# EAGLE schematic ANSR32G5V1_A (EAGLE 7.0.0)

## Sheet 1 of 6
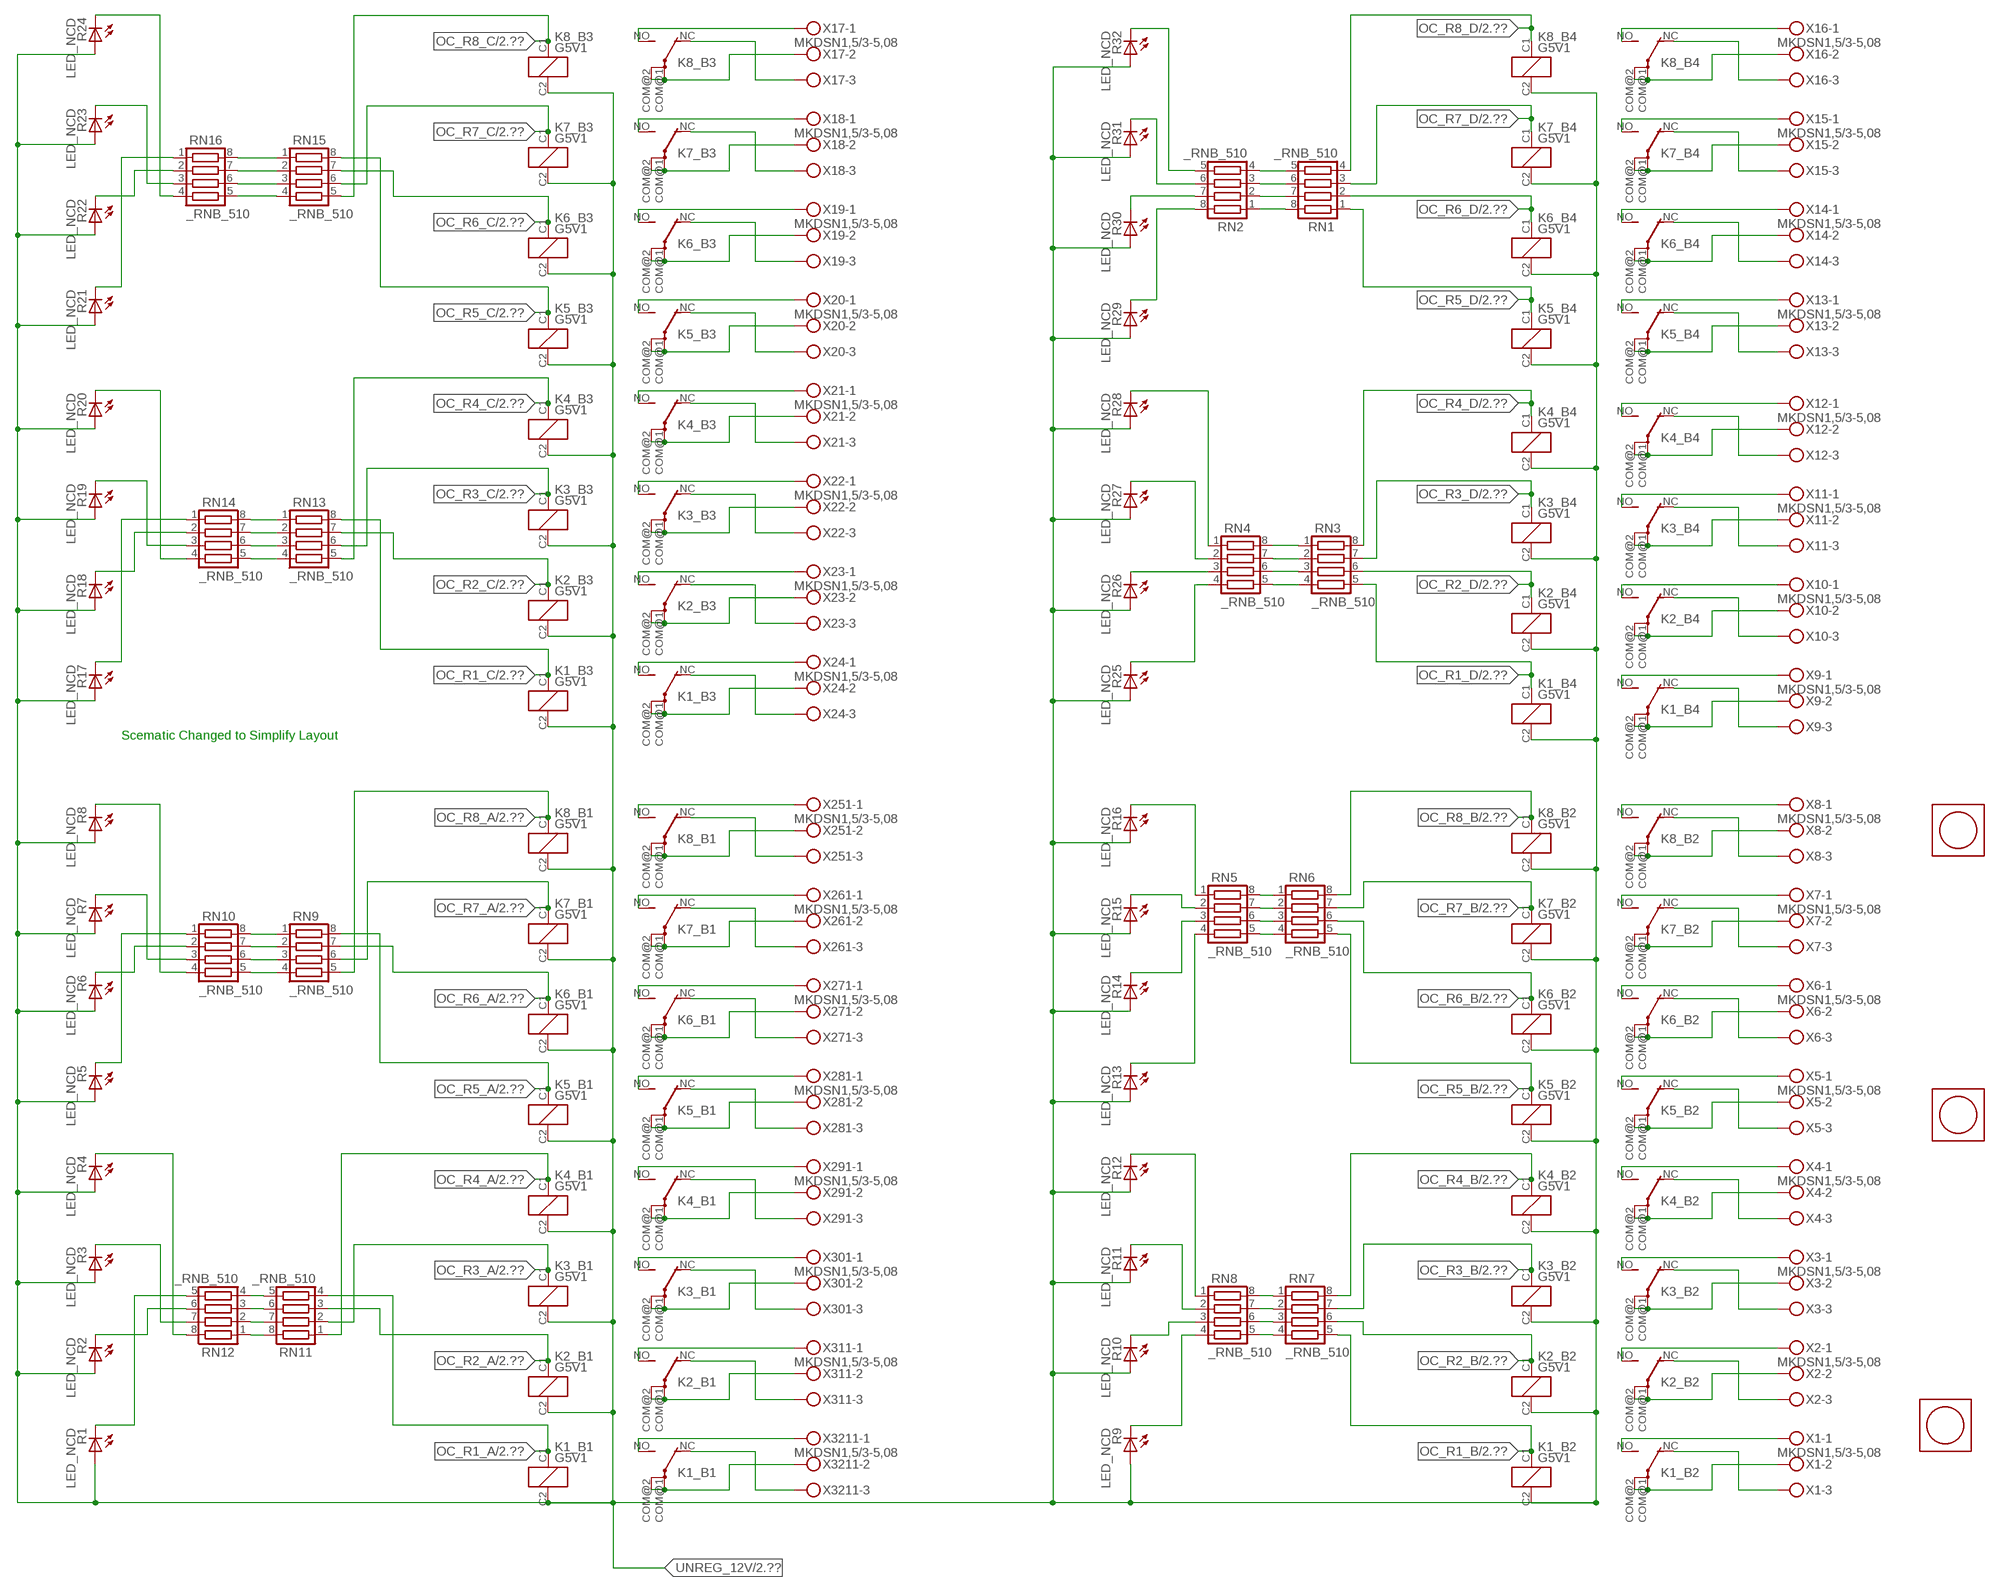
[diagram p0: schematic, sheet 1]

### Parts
K1_B1  G5V1  [G5V1]
K1_B2  G5V1  [G5V1]
K1_B3  G5V1  [G5V1]
K1_B4  G5V1  [G5V1]
K2_B1  G5V1  [G5V1]
K2_B2  G5V1  [G5V1]
K2_B3  G5V1  [G5V1]
K2_B4  G5V1  [G5V1]
K3_B1  G5V1  [G5V1]
K3_B2  G5V1  [G5V1]
K3_B3  G5V1  [G5V1]
K3_B4  G5V1  [G5V1]
K4_B1  G5V1  [G5V1]
K4_B2  G5V1  [G5V1]
K4_B3  G5V1  [G5V1]
K4_B4  G5V1  [G5V1]
K5_B1  G5V1  [G5V1]
K5_B2  G5V1  [G5V1]
K5_B3  G5V1  [G5V1]
K5_B4  G5V1  [G5V1]
K6_B1  G5V1  [G5V1]
K6_B2  G5V1  [G5V1]
K6_B3  G5V1  [G5V1]
K6_B4  G5V1  [G5V1]
K7_B1  G5V1  [G5V1]
K7_B2  G5V1  [G5V1]
K7_B3  G5V1  [G5V1]
K7_B4  G5V1  [G5V1]
K8_B1  G5V1  [G5V1]
K8_B2  G5V1  [G5V1]
K8_B3  G5V1  [G5V1]
K8_B4  G5V1  [G5V1]
R1  LED_NCD  [CHIPLED_0603]
R2  LED_NCD  [CHIPLED_0603]
R3  LED_NCD  [CHIPLED_0603]
R4  LED_NCD  [CHIPLED_0603]
R5  LED_NCD  [CHIPLED_0603]
R6  LED_NCD  [CHIPLED_0603]
R7  LED_NCD  [CHIPLED_0603]
R8  LED_NCD  [CHIPLED_0603]
R9  LED_NCD  [CHIPLED_0603]
R10  LED_NCD  [CHIPLED_0603]
R11  LED_NCD  [CHIPLED_0603]
R12  LED_NCD  [CHIPLED_0603]
R13  LED_NCD  [CHIPLED_0603]
R14  LED_NCD  [CHIPLED_0603]
R15  LED_NCD  [CHIPLED_0603]
R16  LED_NCD  [CHIPLED_0603]
R17  LED_NCD  [CHIPLED_0603]
R18  LED_NCD  [CHIPLED_0603]
R19  LED_NCD  [CHIPLED_0603]
R20  LED_NCD  [CHIPLED_0603]
R21  LED_NCD  [CHIPLED_0603]
R22  LED_NCD  [CHIPLED_0603]
R23  LED_NCD  [CHIPLED_0603]
R24  LED_NCD  [CHIPLED_0603]
R25  LED_NCD  [CHIPLED_0603]
R26  LED_NCD  [CHIPLED_0603]
R27  LED_NCD  [CHIPLED_0603]
R28  LED_NCD  [CHIPLED_0603]
R29  LED_NCD  [CHIPLED_0603]
R30  LED_NCD  [CHIPLED_0603]
R31  LED_NCD  [CHIPLED_0603]
R32  LED_NCD  [CHIPLED_0603]
RN1  _RNB_510  [RNB]
RN2  _RNB_510  [RNB]
RN3  _RNB_510  [RNB]
RN4  _RNB_510  [RNB]
RN5  _RNB_510  [RNB]
RN6  _RNB_510  [RNB]
RN7  _RNB_510  [RNB]
RN8  _RNB_510  [RNB]
RN9  _RNB_510  [RNB]
RN10  _RNB_510  [RNB]
RN11  _RNB_510  [RNB]
RN12  _RNB_510  [RNB]
RN13  _RNB_510  [RNB]
RN14  _RNB_510  [RNB]
RN15  _RNB_510  [RNB]
RN16  _RNB_510  [RNB]
U$1  PCB_MOUNTING_HOLE  [PCB_MOUNTING_HOLE]
U$2  PCB_MOUNTING_HOLE  [PCB_MOUNTING_HOLE]
U$3  PCB_MOUNTING_HOLE  [PCB_MOUNTING_HOLE]
X1  MKDSN1,5/3-5,08  [MKDSN1,5/3-5,08]
X2  MKDSN1,5/3-5,08  [MKDSN1,5/3-5,08]
X3  MKDSN1,5/3-5,08  [MKDSN1,5/3-5,08]
X4  MKDSN1,5/3-5,08  [MKDSN1,5/3-5,08]
X5  MKDSN1,5/3-5,08  [MKDSN1,5/3-5,08]
X6  MKDSN1,5/3-5,08  [MKDSN1,5/3-5,08]
X7  MKDSN1,5/3-5,08  [MKDSN1,5/3-5,08]
X8  MKDSN1,5/3-5,08  [MKDSN1,5/3-5,08]
X9  MKDSN1,5/3-5,08  [MKDSN1,5/3-5,08]
X10  MKDSN1,5/3-5,08  [MKDSN1,5/3-5,08]
X11  MKDSN1,5/3-5,08  [MKDSN1,5/3-5,08]
X12  MKDSN1,5/3-5,08  [MKDSN1,5/3-5,08]
X13  MKDSN1,5/3-5,08  [MKDSN1,5/3-5,08]
X14  MKDSN1,5/3-5,08  [MKDSN1,5/3-5,08]
X15  MKDSN1,5/3-5,08  [MKDSN1,5/3-5,08]
X16  MKDSN1,5/3-5,08  [MKDSN1,5/3-5,08]
X17  MKDSN1,5/3-5,08  [MKDSN1,5/3-5,08]
X18  MKDSN1,5/3-5,08  [MKDSN1,5/3-5,08]
X19  MKDSN1,5/3-5,08  [MKDSN1,5/3-5,08]
X20  MKDSN1,5/3-5,08  [MKDSN1,5/3-5,08]
X21  MKDSN1,5/3-5,08  [MKDSN1,5/3-5,08]
X22  MKDSN1,5/3-5,08  [MKDSN1,5/3-5,08]
X23  MKDSN1,5/3-5,08  [MKDSN1,5/3-5,08]
X24  MKDSN1,5/3-5,08  [MKDSN1,5/3-5,08]
X251  MKDSN1,5/3-5,08  [MKDSN1,5/3-5,08]
X261  MKDSN1,5/3-5,08  [MKDSN1,5/3-5,08]
X271  MKDSN1,5/3-5,08  [MKDSN1,5/3-5,08]
X281  MKDSN1,5/3-5,08  [MKDSN1,5/3-5,08]
X291  MKDSN1,5/3-5,08  [MKDSN1,5/3-5,08]
X301  MKDSN1,5/3-5,08  [MKDSN1,5/3-5,08]
X311  MKDSN1,5/3-5,08  [MKDSN1,5/3-5,08]
X3211  MKDSN1,5/3-5,08  [MKDSN1,5/3-5,08]

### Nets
N$1: K8_B2.COM@1(2:P) K8_B2.COM@2(2:P) X8.2
N$2: K8_B2.NC(2:O) X8.3
N$3: K8_B2.NO(2:S) X8.1
N$4: K7_B2.NO(2:S) X7.1
N$5: K6_B2.NO(2:S) X6.1
N$6: K7_B2.NC(2:O) X7.3
N$7: K7_B2.COM@1(2:P) K7_B2.COM@2(2:P) X7.2
N$8: K6_B2.NC(2:O) X6.3
N$10: K4_B2.NO(2:S) X4.1
N$11: K4_B2.NC(2:O) X4.3
N$12: K4_B2.COM@1(2:P) K4_B2.COM@2(2:P) X4.2
N$14: K6_B2.COM@1(2:P) K6_B2.COM@2(2:P) X6.2
N$33: K5_B2.NC(2:O) X5.3
N$34: K5_B2.COM@1(2:P) K5_B2.COM@2(2:P) X5.2
N$35: K5_B2.NO(2:S) X5.1
N$36: K3_B2.NO(2:S) X3.1
N$37: K3_B2.NC(2:O) X3.3
N$38: K3_B2.COM@1(2:P) K3_B2.COM@2(2:P) X3.2
N$39: K2_B2.NO(2:S) X2.1
N$40: K2_B2.NC(2:O) X2.3
N$41: K2_B2.COM@1(2:P) K2_B2.COM@2(2:P) X2.2
N$42: K1_B2.NO(2:S) X1.1
N$43: K1_B2.NC(2:O) X1.3
N$44: K1_B2.COM@1(2:P) K1_B2.COM@2(2:P) X1.2
N$78: K1_B4.COM@1(2:P) K1_B4.COM@2(2:P) X9.2
N$79: K1_B4.NC(2:O) X9.3
N$80: K1_B4.NO(2:S) X9.1
N$81: K2_B4.NO(2:S) X10.1
N$82: K3_B4.NO(2:S) X11.1
N$83: K2_B4.NC(2:O) X10.3
N$84: K2_B4.COM@1(2:P) K2_B4.COM@2(2:P) X10.2
N$85: K3_B4.NC(2:O) X11.3
N$86: K3_B4.COM@1(2:P) K3_B4.COM@2(2:P) X11.2
N$87: K4_B4.NC(2:O) X12.3
N$88: K4_B4.COM@1(2:P) K4_B4.COM@2(2:P) X12.2
N$89: K4_B4.NO(2:S) X12.1
N$90: K5_B4.NO(2:S) X13.1
N$91: K5_B4.NC(2:O) X13.3
N$92: K5_B4.COM@1(2:P) K5_B4.COM@2(2:P) X13.2
N$93: K6_B4.NO(2:S) X14.1
N$94: K6_B4.NC(2:O) X14.3
N$95: K6_B4.COM@1(2:P) K6_B4.COM@2(2:P) X14.2
N$96: K7_B4.NO(2:S) X15.1
N$97: K7_B4.NC(2:O) X15.3
N$98: K7_B4.COM@1(2:P) K7_B4.COM@2(2:P) X15.2
N$99: K8_B4.NO(2:S) X16.1
N$100: K8_B4.NC(2:O) X16.3
N$101: K8_B4.COM@1(2:P) K8_B4.COM@2(2:P) X16.2
N$179: K8_B3.COM@1(2:P) K8_B3.COM@2(2:P) X17.2
N$180: K8_B3.NC(2:O) X17.3
N$181: K8_B3.NO(2:S) X17.1
N$182: K7_B3.NO(2:S) X18.1
N$183: K6_B3.NO(2:S) X19.1
N$184: K7_B3.NC(2:O) X18.3
N$185: K7_B3.COM@1(2:P) K7_B3.COM@2(2:P) X18.2
N$186: K6_B3.NC(2:O) X19.3
N$187: K6_B3.COM@1(2:P) K6_B3.COM@2(2:P) X19.2
N$188: K5_B3.NC(2:O) X20.3
N$189: K5_B3.COM@1(2:P) K5_B3.COM@2(2:P) X20.2
N$190: K5_B3.NO(2:S) X20.1
N$191: K4_B3.NO(2:S) X21.1
N$192: K4_B3.NC(2:O) X21.3
N$193: K4_B3.COM@1(2:P) K4_B3.COM@2(2:P) X21.2
N$194: K3_B3.NO(2:S) X22.1
N$195: K3_B3.NC(2:O) X22.3
N$196: K3_B3.COM@1(2:P) K3_B3.COM@2(2:P) X22.2
N$197: K2_B3.NO(2:S) X23.1
N$198: K2_B3.NC(2:O) X23.3
N$199: K2_B3.COM@1(2:P) K2_B3.COM@2(2:P) X23.2
N$200: K1_B3.NO(2:S) X24.1
N$201: K1_B3.NC(2:O) X24.3
N$202: K1_B3.COM@1(2:P) K1_B3.COM@2(2:P) X24.2
N$203: K8_B1.COM@1(2:P) K8_B1.COM@2(2:P) X251.2
N$204: K8_B1.NC(2:O) X251.3
N$205: K8_B1.NO(2:S) X251.1
N$206: K7_B1.NO(2:S) X261.1
N$207: K6_B1.NO(2:S) X271.1
N$208: K7_B1.NC(2:O) X261.3
N$209: K7_B1.COM@1(2:P) K7_B1.COM@2(2:P) X261.2
N$210: K6_B1.NC(2:O) X271.3
N$211: K6_B1.COM@1(2:P) K6_B1.COM@2(2:P) X271.2
N$212: K5_B1.NC(2:O) X281.3
N$213: K5_B1.COM@1(2:P) K5_B1.COM@2(2:P) X281.2
N$214: K5_B1.NO(2:S) X281.1
N$215: K4_B1.NO(2:S) X291.1
N$216: K4_B1.NC(2:O) X291.3
N$217: K4_B1.COM@1(2:P) K4_B1.COM@2(2:P) X291.2
N$218: K3_B1.NO(2:S) X301.1
N$219: K3_B1.NC(2:O) X301.3
N$220: K3_B1.COM@1(2:P) K3_B1.COM@2(2:P) X301.2
N$221: K2_B1.NO(2:S) X311.1
N$222: K2_B1.NC(2:O) X311.3
N$223: K2_B1.COM@1(2:P) K2_B1.COM@2(2:P) X311.2
N$224: K1_B1.NO(2:S) X3211.1
N$225: K1_B1.NC(2:O) X3211.3
N$226: K1_B1.COM@1(2:P) K1_B1.COM@2(2:P) X3211.2
N$440: R30.C RN2.7
N$441: R16.C RN5.1
N$442: RN7.2 RN8.7
N$443: RN7.3 RN8.6
N$444: RN7.4 RN8.5
N$445: R15.C RN5.2
N$446: R26.C RN4.3
N$447: R13.C RN5.4
N$448: RN5.5 RN6.4
N$449: RN7.1 RN8.8
N$450: R12.C RN8.1
N$451: RN5.6 RN6.3
N$452: R11.C RN8.2
N$453: RN5.7 RN6.2
N$454: RN5.8 RN6.1
N$455: RN3.4 RN4.5
N$456: R32.C RN2.5
N$458: R14.C RN5.3
N$459: R10.C RN8.3
N$460: R29.C RN2.8
N$461: R28.C RN4.1
N$462: R27.C RN4.2
N$463: RN11.5 RN12.4
N$464: R25.C RN4.4
N$465: RN1.8 RN2.1
N$466: RN1.7 RN2.2
N$467: RN1.6 RN2.3
N$468: RN1.5 RN2.4
N$469: R31.C RN2.6
N$470: R9.C RN8.4
N$473: R1.C RN12.5
N$474: RN11.6 RN12.3
N$475: R2.C RN12.6
N$476: R3.C RN12.7
N$477: RN9.4 RN10.5
N$478: RN9.3 RN10.6
N$479: RN9.2 RN10.7
N$480: RN9.1 RN10.8
N$481: RN11.7 RN12.2
N$482: R5.C RN10.1
N$483: R4.C RN12.8
N$484: R7.C RN10.3
N$485: R8.C RN10.4
N$486: R6.C RN10.2
N$487: R19.C RN14.3
N$488: R18.C RN14.2
N$489: R17.C RN14.1
N$490: R24.C RN16.4
N$491: RN15.3 RN16.6
N$492: RN15.2 RN16.7
N$493: RN15.1 RN16.8
N$494: R20.C RN14.4
N$495: R23.C RN16.3
N$496: R22.C RN16.2
N$497: R21.C RN16.1
N$500: RN11.8 RN12.1
N$501: RN13.4 RN14.5
N$502: RN13.3 RN14.6
N$503: RN13.2 RN14.7
N$504: RN13.1 RN14.8
N$505: RN3.3 RN4.6
N$506: RN3.2 RN4.7
N$507: RN3.1 RN4.8
N$514: RN15.4 RN16.5
OC_R1_A: K1_B1.C1(1:C1) RN11.4 ; also sheet 2
OC_R1_B: K1_B2.C1(1:C1) RN7.5 ; also sheet 2
OC_R1_C: K1_B3.C1(1:C1) RN13.8 ; also sheet 2
OC_R1_D: K1_B4.C1(1:C1) RN3.5 ; also sheet 2
OC_R2_A: K2_B1.C1(1:C1) RN11.3 ; also sheet 2
OC_R2_B: K2_B2.C1(1:C1) RN7.6 ; also sheet 2
OC_R2_C: K2_B3.C1(1:C1) RN13.7 ; also sheet 2
OC_R2_D: K2_B4.C1(1:C1) RN3.6 ; also sheet 2
OC_R3_A: K3_B1.C1(1:C1) RN11.2 ; also sheet 2
OC_R3_B: K3_B2.C1(1:C1) RN7.7 ; also sheet 2
OC_R3_C: K3_B3.C1(1:C1) RN13.6 ; also sheet 2
OC_R3_D: K3_B4.C1(1:C1) RN3.7 ; also sheet 2
OC_R4_A: K4_B1.C1(1:C1) RN11.1 ; also sheet 2
OC_R4_B: K4_B2.C1(1:C1) RN7.8 ; also sheet 2
OC_R4_C: K4_B3.C1(1:C1) RN13.5 ; also sheet 2
OC_R4_D: K4_B4.C1(1:C1) RN3.8 ; also sheet 2
OC_R5_A: K5_B1.C1(1:C1) RN9.8 ; also sheet 2
OC_R5_B: K5_B2.C1(1:C1) RN6.5 ; also sheet 2
OC_R5_C: K5_B3.C1(1:C1) RN15.8 ; also sheet 2
OC_R5_D: K5_B4.C1(1:C1) RN1.1 ; also sheet 2
OC_R6_A: K6_B1.C1(1:C1) RN9.7 ; also sheet 2
OC_R6_B: K6_B2.C1(1:C1) RN6.6 ; also sheet 2
OC_R6_C: K6_B3.C1(1:C1) RN15.7 ; also sheet 2
OC_R6_D: K6_B4.C1(1:C1) RN1.2 ; also sheet 2
OC_R7_A: K7_B1.C1(1:C1) RN9.6 ; also sheet 2
OC_R7_B: K7_B2.C1(1:C1) RN6.7 ; also sheet 2
OC_R7_C: K7_B3.C1(1:C1) RN15.6 ; also sheet 2
OC_R7_D: K7_B4.C1(1:C1) RN1.3 ; also sheet 2
OC_R8_A: K8_B1.C1(1:C1) RN9.5 ; also sheet 2
OC_R8_B: K8_B2.C1(1:C1) RN6.8 ; also sheet 2
OC_R8_C: K8_B3.C1(1:C1) RN15.5 ; also sheet 2
OC_R8_D: K8_B4.C1(1:C1) RN1.4 ; also sheet 2
UNREG_12V: K1_B1.C2(1:C2) K1_B2.C2(1:C2) K1_B3.C2(1:C2) K1_B4.C2(1:C2) K2_B1.C2(1:C2) K2_B2.C2(1:C2) K2_B3.C2(1:C2) K2_B4.C2(1:C2) K3_B1.C2(1:C2) K3_B2.C2(1:C2) K3_B3.C2(1:C2) K3_B4.C2(1:C2) K4_B1.C2(1:C2) K4_B2.C2(1:C2) K4_B3.C2(1:C2) K4_B4.C2(1:C2) K5_B1.C2(1:C2) K5_B2.C2(1:C2) K5_B3.C2(1:C2) K5_B4.C2(1:C2) K6_B1.C2(1:C2) K6_B2.C2(1:C2) K6_B3.C2(1:C2) K6_B4.C2(1:C2) K7_B1.C2(1:C2) K7_B2.C2(1:C2) K7_B3.C2(1:C2) K7_B4.C2(1:C2) K8_B1.C2(1:C2) K8_B2.C2(1:C2) K8_B3.C2(1:C2) K8_B4.C2(1:C2) R1.A R2.A R3.A R4.A R5.A R6.A R7.A R8.A R9.A R10.A R11.A R12.A R13.A R14.A R15.A R16.A R17.A R18.A R19.A R20.A R21.A R22.A R23.A R24.A R25.A R26.A R27.A R28.A R29.A R30.A R31.A R32.A ; also sheet 2,3

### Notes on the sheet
- Scematic Changed to Simplify Layout

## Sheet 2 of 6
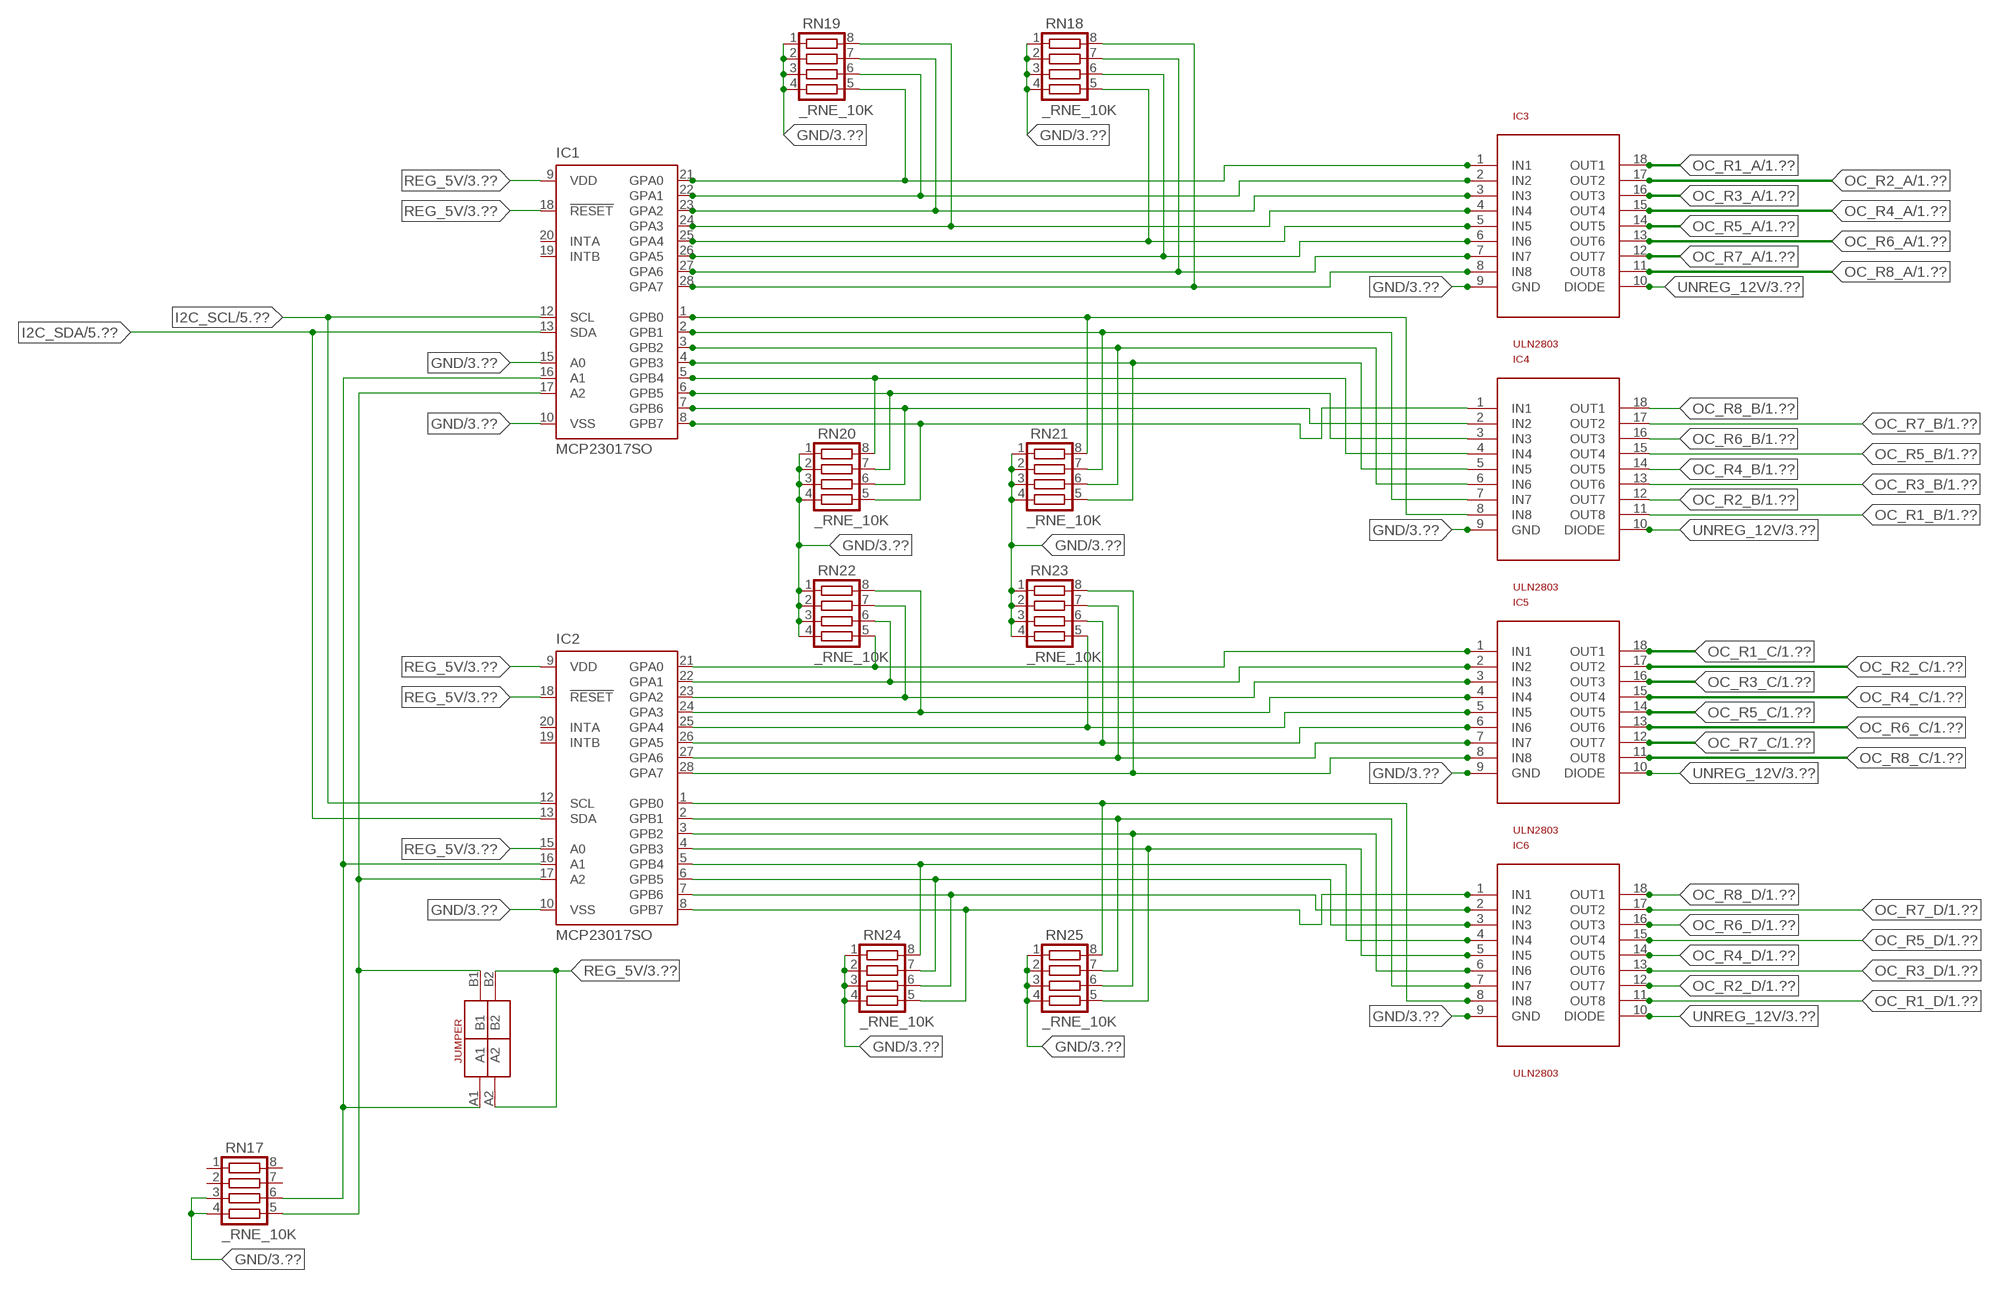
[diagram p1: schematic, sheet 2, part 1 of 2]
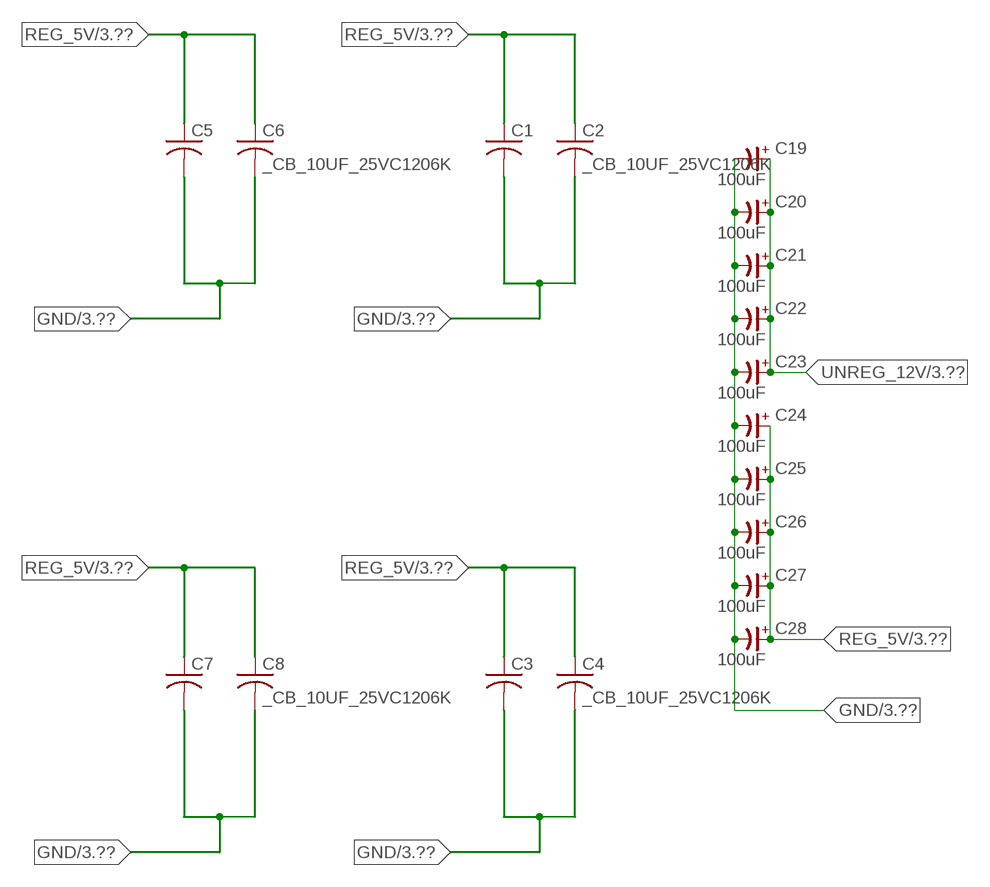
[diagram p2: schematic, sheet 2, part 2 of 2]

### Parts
C1  _CA_.10UF_50VC1206K  [_CA_.1UF_50V]
C2  _CB_10UF_25VC1206K  [_CB_10UF_25V]
C3  _CA_.10UF_50VC1206K  [_CA_.1UF_50V]
C4  _CB_10UF_25VC1206K  [_CB_10UF_25V]
C5  _CA_.10UF_50VC1206K  [_CA_.1UF_50V]
C6  _CB_10UF_25VC1206K  [_CB_10UF_25V]
C7  _CA_.10UF_50VC1206K  [_CA_.1UF_50V]
C8  _CB_10UF_25VC1206K  [_CB_10UF_25V]
C19  100uF  CP-E-025X060  [E-025X060]
C20  100uF  CP-E-025X060  [E-025X060]
C21  100uF  CP-E-025X060  [E-025X060]
C22  100uF  CP-E-025X060  [E-025X060]
C23  100uF  CP-E-025X060  [E-025X060]
C24  100uF  CP-E-025X060  [E-025X060]
C25  100uF  CP-E-025X060  [E-025X060]
C26  100uF  CP-E-025X060  [E-025X060]
C27  100uF  CP-E-025X060  [E-025X060]
C28  100uF  CP-E-025X060  [E-025X060]
IC1  MCP23017SO  [SO28W]
IC2  MCP23017SO  [SO28W]
IC3  ULN2803  [SO18L]
IC4  ULN2803  [SO18L]
IC5  ULN2803  [SO18L]
IC6  ULN2803  [SO18L]
RN17  _RNE_10K  [RNE]
RN18  _RNE_10K  [RNE]
RN19  _RNE_10K  [RNE]
RN20  _RNE_10K  [RNE]
RN21  _RNE_10K  [RNE]
RN22  _RNE_10K  [RNE]
RN23  _RNE_10K  [RNE]
RN24  _RNE_10K  [RNE]
RN25  _RNE_10K  [RNE]
U$13  JUMPER_2X2  [JUMPER_2X2]

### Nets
GND: C1.2 C2.2 C3.2 C4.2 C5.2 C6.2 C7.2 C8.2 C19.- C20.- C21.- C22.- C23.- C24.- C25.- C26.- C27.- C28.- IC1.10(VSS) IC1.15(A0) IC2.10(VSS) IC3.9(GND) IC4.9(GND) IC5.9(GND) IC6.9(GND) RN17.3 RN17.4 RN18.1 RN18.2 RN18.3 RN18.4 RN19.1 RN19.2 RN19.3 RN19.4 RN20.1 RN20.2 RN20.3 RN20.4 RN21.1 RN21.2 RN21.3 RN21.4 RN22.1 RN22.2 RN22.3 RN22.4 RN23.1 RN23.2 RN23.3 RN23.4 RN24.1 RN24.2 RN24.3 RN24.4 RN25.1 RN25.2 RN25.3 RN25.4 ; also sheet 3,4,5,6
I2C_SCL: IC1.12(SCL) IC2.12(SCL) ; also sheet 5,6
I2C_SDA: IC1.13(SDA) IC2.13(SDA) ; also sheet 5,6
N$405: IC1.21(GPA0) IC3.1(IN1) RN19.5
N$406: IC1.25(GPA4) IC3.5(IN5) RN18.5
N$407: IC1.26(GPA5) IC3.6(IN6) RN18.6
N$408: IC1.16(A1) IC2.16(A1) RN17.6 U$13.A1
N$409: IC1.22(GPA1) IC3.2(IN2) RN19.6
N$410: IC1.23(GPA2) IC3.3(IN3) RN19.7
N$411: IC1.24(GPA3) IC3.4(IN4) RN19.8
N$416: IC1.1(GPB0) IC4.8(IN8) RN21.8
N$417: IC1.2(GPB1) IC4.7(IN7) RN21.7
N$418: IC1.3(GPB2) IC4.6(IN6) RN21.6
N$419: IC1.4(GPB3) IC4.5(IN5) RN21.5
N$420: IC1.5(GPB4) IC4.4(IN4) RN20.8
N$421: IC1.6(GPB5) IC4.3(IN3) RN20.7
N$422: IC1.7(GPB6) IC4.2(IN2) RN20.6
N$423: IC1.8(GPB7) IC4.1(IN1) RN20.5
N$424: IC2.21(GPA0) IC5.1(IN1) RN22.5
N$425: IC2.22(GPA1) IC5.2(IN2) RN22.6
N$426: IC2.23(GPA2) IC5.3(IN3) RN22.7
N$427: IC2.24(GPA3) IC5.4(IN4) RN22.8
N$428: IC2.25(GPA4) IC5.5(IN5) RN23.5
N$429: IC2.26(GPA5) IC5.6(IN6) RN23.6
N$430: IC2.27(GPA6) IC5.7(IN7) RN23.7
N$431: IC2.28(GPA7) IC5.8(IN8) RN23.8
N$432: IC2.1(GPB0) IC6.8(IN8) RN25.8
N$433: IC2.2(GPB1) IC6.7(IN7) RN25.7
N$434: IC2.3(GPB2) IC6.6(IN6) RN25.6
N$435: IC2.4(GPB3) IC6.5(IN5) RN25.5
N$436: IC2.5(GPB4) IC6.4(IN4) RN24.8
N$437: IC2.6(GPB5) IC6.3(IN3) RN24.7
N$438: IC2.7(GPB6) IC6.2(IN2) RN24.6
N$439: IC2.8(GPB7) IC6.1(IN1) RN24.5
N$498: IC1.17(A2) IC2.17(A2) RN17.5 U$13.B1
N$525: IC1.27(GPA6) IC3.7(IN7) RN18.7
N$526: IC1.28(GPA7) IC3.8(IN8) RN18.8
OC_R1_A: IC3.18(OUT1) ; also sheet 1
OC_R1_B: IC4.11(OUT8) ; also sheet 1
OC_R1_C: IC5.18(OUT1) ; also sheet 1
OC_R1_D: IC6.11(OUT8) ; also sheet 1
OC_R2_A: IC3.17(OUT2) ; also sheet 1
OC_R2_B: IC4.12(OUT7) ; also sheet 1
OC_R2_C: IC5.17(OUT2) ; also sheet 1
OC_R2_D: IC6.12(OUT7) ; also sheet 1
OC_R3_A: IC3.16(OUT3) ; also sheet 1
OC_R3_B: IC4.13(OUT6) ; also sheet 1
OC_R3_C: IC5.16(OUT3) ; also sheet 1
OC_R3_D: IC6.13(OUT6) ; also sheet 1
OC_R4_A: IC3.15(OUT4) ; also sheet 1
OC_R4_B: IC4.14(OUT5) ; also sheet 1
OC_R4_C: IC5.15(OUT4) ; also sheet 1
OC_R4_D: IC6.14(OUT5) ; also sheet 1
OC_R5_A: IC3.14(OUT5) ; also sheet 1
OC_R5_B: IC4.15(OUT4) ; also sheet 1
OC_R5_C: IC5.14(OUT5) ; also sheet 1
OC_R5_D: IC6.15(OUT4) ; also sheet 1
OC_R6_A: IC3.13(OUT6) ; also sheet 1
OC_R6_B: IC4.16(OUT3) ; also sheet 1
OC_R6_C: IC5.13(OUT6) ; also sheet 1
OC_R6_D: IC6.16(OUT3) ; also sheet 1
OC_R7_A: IC3.12(OUT7) ; also sheet 1
OC_R7_B: IC4.17(OUT2) ; also sheet 1
OC_R7_C: IC5.12(OUT7) ; also sheet 1
OC_R7_D: IC6.17(OUT2) ; also sheet 1
OC_R8_A: IC3.11(OUT8) ; also sheet 1
OC_R8_B: IC4.18(OUT1) ; also sheet 1
OC_R8_C: IC5.11(OUT8) ; also sheet 1
OC_R8_D: IC6.18(OUT1) ; also sheet 1
REG_5V: C1.1 C2.1 C3.1 C4.1 C5.1 C6.1 C7.1 C8.1 C24.+ C25.+ C26.+ C27.+ C28.+ IC1.9(VDD) IC1.18(!RESET) IC2.9(VDD) IC2.15(A0) IC2.18(!RESET) U$13.A2 U$13.B2 ; also sheet 3,4,5,6
UNREG_12V: C19.+ C20.+ C21.+ C22.+ C23.+ IC3.10(DIODE) IC4.10(DIODE) IC5.10(DIODE) IC6.10(DIODE) ; also sheet 1,3
Unconnected: IC1.19(INTB) IC1.20(INTA) IC2.19(INTB) IC2.20(INTA) RN17.1 RN17.2 RN17.7 RN17.8

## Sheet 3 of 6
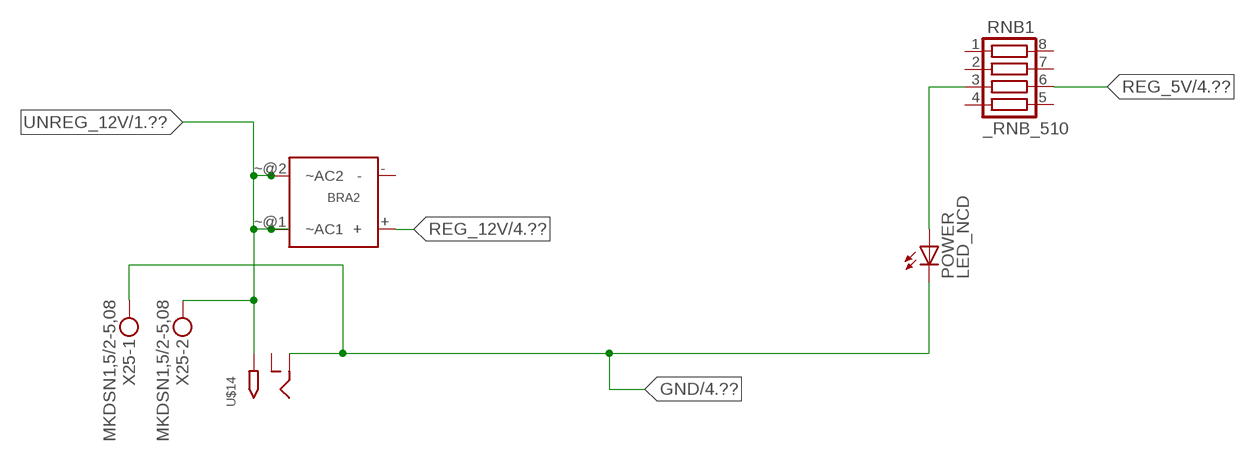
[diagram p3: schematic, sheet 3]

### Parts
BRA2  MB2S_  [MB2S]
POWER  LED_NCD  [CHIPLED_0603]
RNB1  _RNB_510  [RNB]
U$14  2.1MMJACK  [PJ-102A]
X25  MKDSN1,5/2-5,08  [MKDSN1,5/2-5,08]

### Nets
GND: POWER.C U$14.RING X25.1 ; also sheet 2,4,5,6
N$9: POWER.A RNB1.3
REG_5V: RNB1.6 ; also sheet 2,4,5,6
REG_12V: BRA2.+ ; also sheet 4
UNREG_12V: BRA2.~@1(~AC1) BRA2.~@2(~AC2) U$14.TIP X25.2 ; also sheet 1,2
Unconnected: BRA2.- RNB1.1 RNB1.2 RNB1.4 RNB1.5 RNB1.7 RNB1.8 U$14.RING_SW

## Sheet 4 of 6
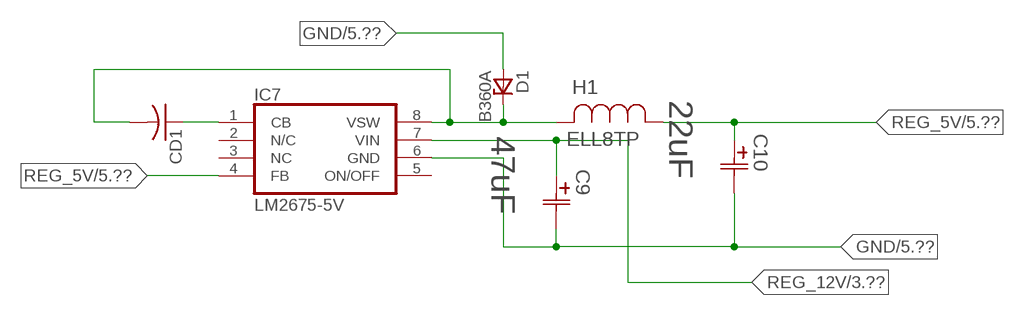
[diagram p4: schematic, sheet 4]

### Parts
C9  47uF  490-5463-6-NDCAP  [C2917(7343)-Y]
C10  22uF  490-5463-6-NDCAP  [C2917(7343)-Y]
CD1  _CD_10NF_50VC1206K  [_CD_10NF_50V]
D1  B360A  [DO214AC_ZENER]
H1  ELL8TP  [IND_ELL8TP]
IC7  LM2675-5V  LM2675  [SO-8]

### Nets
GND: C9.2(C2) C10.2(C2) D1.A IC7.6(GND) ; also sheet 2,3,5,6
N$13: CD1.2 D1.C H1.2 IC7.8(VSW)
N$15: CD1.1 IC7.1(CB)
REG_5V: C10.1(C1) H1.1 IC7.4(FB) ; also sheet 2,3,5,6
REG_12V: C9.1(C1) IC7.7(VIN) ; also sheet 3
Unconnected: IC7.2(N/C) IC7.5(ON/OFF)

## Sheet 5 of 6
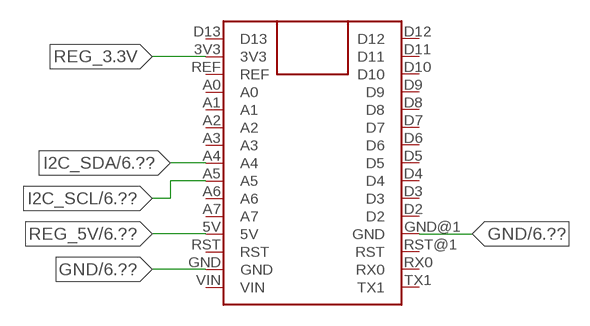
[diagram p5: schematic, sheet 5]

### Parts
FOR_NANO  ARDUINO_NANO  [ARDUINO_NANO]

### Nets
GND: FOR_NANO.GND FOR_NANO.GND@1(GND) ; also sheet 2,3,4,6
I2C_SCL: FOR_NANO.A5 ; also sheet 2,6
I2C_SDA: FOR_NANO.A4 ; also sheet 2,6
REG_3.3V: FOR_NANO.3V3
REG_5V: FOR_NANO.5V ; also sheet 2,3,4,6
Unconnected: FOR_NANO.A0 FOR_NANO.A1 FOR_NANO.A2 FOR_NANO.A3 FOR_NANO.A6 FOR_NANO.A7 FOR_NANO.D2 FOR_NANO.D3 FOR_NANO.D4 FOR_NANO.D5 FOR_NANO.D6 FOR_NANO.D7 FOR_NANO.D8 FOR_NANO.D9 FOR_NANO.D10 FOR_NANO.D11 FOR_NANO.D12 FOR_NANO.D13 FOR_NANO.REF FOR_NANO.RST FOR_NANO.RST@1(RST) FOR_NANO.RX0 FOR_NANO.TX1 FOR_NANO.VIN

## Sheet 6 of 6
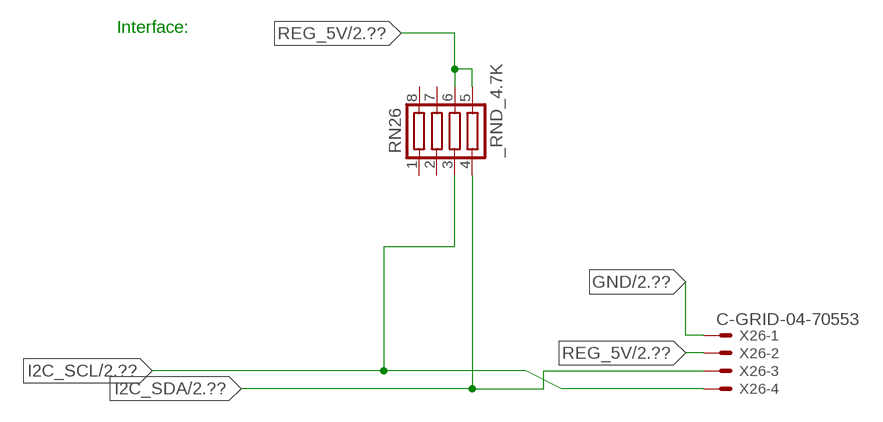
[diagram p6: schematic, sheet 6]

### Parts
RN26  _RND_4.7K  [RND]
X26  C-GRID-04-70553  [70553-04]

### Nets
GND: X26.1 ; also sheet 2,3,4,5
I2C_SCL: RN26.3 X26.4 ; also sheet 2,5
I2C_SDA: RN26.4 X26.3 ; also sheet 2,5
REG_5V: RN26.5 RN26.6 X26.2 ; also sheet 2,3,4,5
Unconnected: RN26.1 RN26.2 RN26.7 RN26.8

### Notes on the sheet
- Interface:

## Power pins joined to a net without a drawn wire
NC: IC7.3(NC)

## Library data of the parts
BRA2 = NCD_ULTIMATE_LIBRARY:MB2S: Bridge Rectifier BRA MB2S 200V 500ma Digikey MB2S-TPMSTR-ND/MB2S-TP
C1 C3 C5 C7 = NCD_ULTIMATE_LIBRARY:_CA_.10UF_50V: Capacitor .1uF SMT
C2 C4 C6 C8 = NCD_ULTIMATE_LIBRARY:_CB_10UF_25V: Capacitor 10uF SMT
C9 C10 = NCD_ULTIMATE_bhaskar:490-5463-6-ND: NCD CAP
C19-C28 = NCD_ULTIMATE_LIBRARY:CP-: Capacitors All Kinds POLARIZED CAP
CD1 = NCD_ULTIMATE_LIBRARY:_CD_10NF_50V: Capacitor 10nF SMT
D1 = NCD_ULTIMATE_bhaskar:B360A: NCD DIODE B350A/B360A
FOR_NANO = NCD_ULTIMATE_CONNECTORS:ARDUINO_NANO
H1 = NCD_ULTIMATE_bhaskar:ELL8TP: NCD coil
IC1 IC2 = NCD_ULTIMATE_LIBRARY:MCP23017: Semiconductor Port Expander I/O 16-Bit I2C http://ww1.microchip.com/downloads/en/DeviceDoc/21952a.pdf Source: http://ww1.microchip.com/downloads/en/DeviceDoc/21952a.pdf
IC3-IC6 = NCD_ULTIMATE_LIBRARY:ULN2803: Semiconductor 8 O.C. N-Channel Transistor Driver Digikey ULN2803AFWGCELTR-ND/ULN2803AFWG,C,EL
IC7 = NCD_ULTIMATE_bhaskar:LM2675: LM2675 NCD http://www.ti.com/lit/ds/symlink/lm2675.pdf
K1_B1-K1_B4 K2_B1-K2_B4 K3_B1-K3_B4 K4_B1-K4_B4 K5_B1-K5_B4 K6_B1-K6_B4 K7_B1-K7_B4 K8_B1-K8_B4 = NCD_ULTIMATE_LIBRARY:G5V1: RELAY 1 x switch, 0.5 A/125 V AC, 1 A/24 V DC , Omron
POWER R1-R32 = NCD_ULTIMATE_bhaskar:LED_NCD
RN1-RN16 RNB1 = NCD_ULTIMATE_LIBRARY:_RNB_510: Resistor Array RNB SMT 510 x 4 Single Resistor Source: http://www.ctscorp.com/components/Datasheets/CTSChipArrayDs.pdf Digikey 742C083511JPTR-ND/ 742C083511JP; OC_FARNELL: unknown; OC_NEWARK: unknown
RN17-RN25 = NCD_ULTIMATE_LIBRARY:_RNE_10K: Resistor Array RNE SMT 10K x 4 Single Resistor Source: http://www.ctscorp.com/components/Datasheets/CTSChipArrayDs.pdf Digikey 742C083103JPTR-ND/742C083103JP; OC_FARNELL: unknown; OC_NEWARK: unknown
RN26 = NCD_ULTIMATE_LIBRARY:_RND_4.7K: Resistor Array RND SMT 4.7K x 4 Single Resistor Source: http://www.ctscorp.com/components/Datasheets/CTSChipArrayDs.pdf Digikey 742C083472JPTR-ND/742C083472JP; OC_FARNELL: unknown; OC_NEWARK: unknown
U$1-U$3 = NCD_ULTIMATE_CONNECTORS:PCB_MOUNTING_HOLE
U$13 = NCD_ULTIMATE_CONNECTORS:JUMPER_2X2
U$14 = NCD_ULTIMATE_CONNECTORS:2.1MMJACK: 2.1mm x 5.5mm DC jack with internal switch. Digikey part #PJ-102A, 4UCON part #05537 By microbuilder.eu
X1-X24 X251 X261 X271 X281 X291 X301 X311 X3211 = NCD_ULTIMATE_CONNECTORS:MKDSN1,5/3-5,08: MKDSN 1,5/ 3-5,08 Printklemme Nennstrom: 13,5 A Nennspannung: 250 V Rastermaß: 5,08 mm Polzahl: 3 Anschlussart: Schraubanschluss Montage: Löten Anschlussrichtung Leiter/Platine: 0 ° Artikelnummer: 1729131 Source: http://eshop.phoenixcontact.com .. 1729131.pdf
X25 = NCD_ULTIMATE_CONNECTORS:MKDSN1,5/2-5,08: MKDSN 1,5/ 2-5,08 Printklemme
X26 = NCD_ULTIMATE_CONNECTORS:C-GRID-04: CONNECTOR 4-Pos I2C wire to board 2.54 mm (0.100") pitch header Digikey WM1342-ND/0015912045; OC_FARNELL: unknown; OC_NEWARK: unknown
